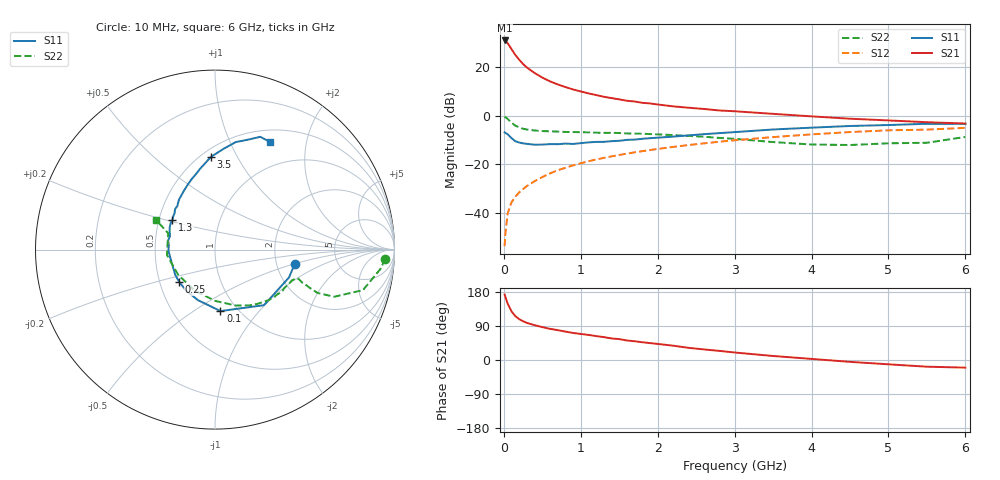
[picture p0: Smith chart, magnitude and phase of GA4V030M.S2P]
! Infineon Technologies  Discrete & RF Semiconductors
! BF775
! Si NPN RF Bipolar Junction Transistor in SOT23
! VCE = 4 V  IC = 30 mA
! Common Emitter S-Parameters:  May  1996
# GHz  S  MA  R  50
!  f  S11  S21  S12  S22
! GHz  MAG  ANG  MAG  ANG  MAG  ANG  MAG  ANG
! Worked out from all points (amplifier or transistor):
!   36 points, 10 MHz to 6 GHz, reference 50 ohm
!   highest |S21| = 30.8 dB at 10 MHz (marker M1)
!   |S21| within 3 dB of that: start of sweep to 88.09 MHz
!   unconditionally stable (mu >= 1): 259.5 MHz to 2.98 GHz
!   at 250 MHz: K = 0.99, MSG = 25.6 dB, |S12| = -30.2 dB
!   at 1.4 GHz: K = 1.15, MAG = 9.6 dB, |S12| = -16.8 dB
!   at 6 GHz: K = 0.98, MSG = 0.9 dB, |S12| = -5.1 dB
!   S11 on the Smith chart (normalised r, x): 10 MHz: 2.52, -0.52; 100 MHz: 0.83, -0.65; 250 MHz: 0.63, -0.25; 1.3 GHz: 0.59, +0.21; 3.5 GHz: 0.56, +0.79; 6 GHz: 0.65, +1.43
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0.01  0.4511 -10.5  34.55 172.9  0.0021 84.5  0.9506 -3.1
0.02  0.4404 -20.7  33.98 166.1  0.0038 82.6  0.9279 -6.7
0.05  0.4128 -48.6  30.32 148.6  0.0099 72.8  0.8549 -15.3
0.1  0.3438 -84.9  22.87 128.2  0.0167 67.3  0.7138 -21.6
0.15  0.2972 -108.7  17.38 115.6  0.0217 66.8  0.6196 -22.9
0.2  0.2794 -124.9  13.89 107.8  0.0266 68.5  0.5712 -22.0
0.25  0.2688 -137.8  11.35 102.2  0.031 69.3  0.5353 -21.0
0.3  0.2625 -147.3  9.635 97.9  0.0359 70.6  0.5168 -20.6
0.4  0.2526 -161.2  7.426 91.9  0.0451 72.1  0.4935 -19.3
0.5  0.2535 -170.7  5.991 86.8  0.0548 73.0  0.4801 -19.3
0.6  0.2597 -178.8  5.016 82.2  0.0651 73.1  0.4742 -19.9
0.8  0.2659 168.8  3.83 75.0  0.0848 72.4  0.4606 -22.0
0.9  0.2616 163.4  3.423 71.4  0.0952 71.8  0.4585 -22.9
1.1  0.2816 153.7  2.84 66.2  0.1155 70.7  0.4522 -26.2
1.3  0.2888 145.3  2.421 60.4  0.1354 69.0  0.4414 -29.3
1.6  0.3171 134.5  2.006 51.5  0.1659 66.2  0.4302 -34.9
2.2  0.369 118.3  1.541 37.8  0.2273 60.1  0.3974 -47.2
2.8  0.4357 103.8  1.269 24.1  0.2903 53.0  0.348 -63.5
3.5  0.5172 92.5  1.082 10.6  0.3615 43.7  0.2857 -90.0
4.5  0.6099 79.1  0.86 -4.9  0.4582 29.5  0.2487 -145.5
5.5  0.6773 68.1  0.729 -17.7  0.5147 13.4  0.2764 160.7
6  0.6732 62.8  0.685 -20.1  0.5579 8.9  0.3642 153.5
